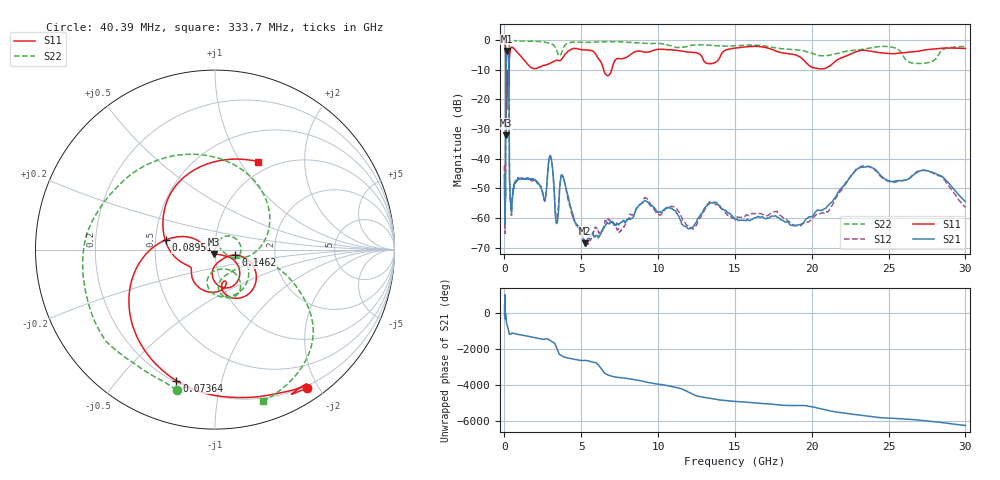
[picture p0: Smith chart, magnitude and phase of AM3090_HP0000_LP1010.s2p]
! Date/Time: Thu, Feb 28, 2019 1:53 PM
! Network Analyzer: Agilent Technologies E8364B Rev: A.07.50.67
! Sweep from 0.010 to 30.000 GHz, 1601 Points, Sweep Type: LOG
! Power Supply: 5.023 V, 0.002 A
# Hz S DB R 50
!freq MagS11 AngS11 MagS21 AngS21 MagS12 AngS12 MagS22 AngS22
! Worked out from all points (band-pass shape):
!   1601 points, 10 MHz to 30 GHz, reference 50 ohm
!   highest |S21| = -3.72 dB at 150.6 MHz (marker M1); lowest = -68.5 dB at 5.232 GHz (marker M2)
!   |S21| within 3 dB of the highest: 99.5 MHz to 270.2 MHz (170.7 MHz wide, 92.3 % of centre)
!   lowest |S11| = -32.1 dB at 97.94 MHz (marker M3), VSWR 1.05, Z = 49.2 - j2.33 ohm
!   |S11| at or under -10 dB: 88.91 MHz to 298.5 MHz (209.6 MHz wide, 108 % of centre); 6.455 GHz to 6.979 GHz (524.2 MHz wide, 7.8 % of centre)
!   |S22| runs from -30.6 to -0.2 dB; largest |S21 - S12| = 0.012
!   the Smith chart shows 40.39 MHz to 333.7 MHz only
!   S11 on the Smith chart (normalised r, x): 40.39 MHz: 0.17, -1.86; 73.64 MHz: 0.21, -0.73; 89.51 MHz: 0.57, +0.07; 146.2 MHz: 1.25, -0.08; 333.7 MHz: 0.86, +1.20
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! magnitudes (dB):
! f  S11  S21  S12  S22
! 10 MHz  -0.3  -50.1  -42.5  -0.7
! 38.04 MHz  -0.5  -59.0  -64.0  -1.6
! 40.39 MHz  -0.7  -60.5  -63.3  -1.8
! 73.64 MHz  -2.4  -47.2  -45.7  -4.4
! 89.51 MHz  -11.1  -15.0  -15.0  -11.3
! 97.94 MHz  -32.1  -7.2  -7.2  -29.3
! 113.8 MHz  -13.2  -4.8  -4.8  -18.7
! 144.7 MHz  -19.9  -3.7  -3.7  -18.5
! 146.2 MHz  -18.6  -3.7  -3.7  -18.2
! 150.6 MHz  -15.3  -3.7  -3.7  -16.7
! 274.6 MHz  -15.1  -7.4  -7.4  -16.2
! 333.7 MHz  -5.3  -47.8  -47.9  -1.0
! 550.5 MHz  -2.7  -50.8  -52.0  -0.3
! 2.084 GHz  -9.6  -47.6  -47.7  -0.5
! 3.002 GHz  -7.8  -39.1  -39.2  -1.2
! 3.385 GHz  -6.8  -61.8  -60.1  -3.3
! 3.798 GHz  -6.0  -45.9  -46.0  -3.2
! 5.232 GHz  -3.3  -68.5  -67.6  -0.8
! 7.926 GHz  -5.9  -61.0  -61.6  -0.7
! 19.31 GHz  -6.0  -62.0  -62.4  -3.4
! 23.48 GHz  -3.5  -42.8  -42.5  -3.0
! 30 GHz  -2.9  -54.4  -56.4  -2.2
